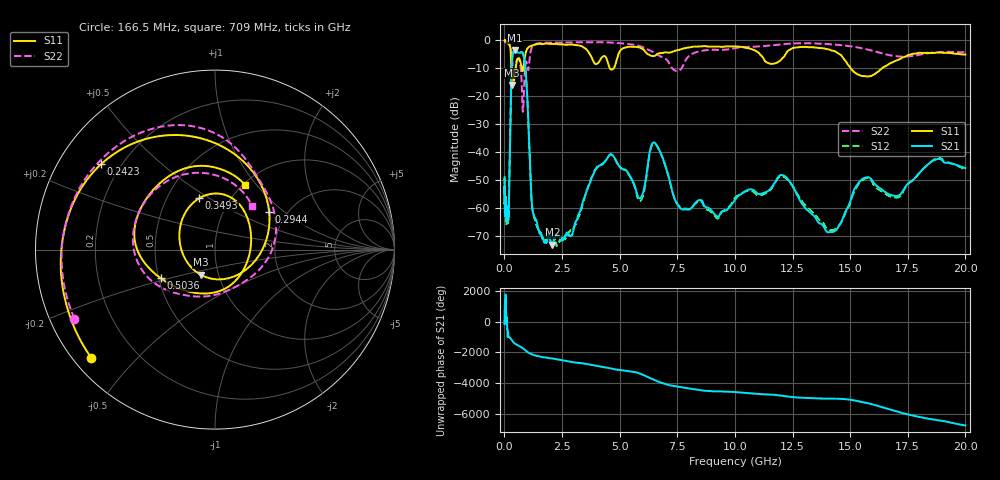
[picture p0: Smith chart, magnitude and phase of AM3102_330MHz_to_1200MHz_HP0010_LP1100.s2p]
! Date/Time: Tue, Sep 11, 2018 5:11 PM
! Network Analyzer: Agilent Technologies E8362B Rev: A.07.50.63
! Sweep from 0.010 to 20.000 GHz, 1601 Points, Sweep Type: LOG
! Power Supply: 4.949 V, 0.001 A
# Hz S DB R 50
!freq MagS11 AngS11 MagS21 AngS21 MagS12 AngS12 MagS22 AngS22
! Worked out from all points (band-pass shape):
!   1601 points, 10 MHz to 20 GHz, reference 50 ohm
!   highest |S21| = -3.37 dB at 458 MHz (marker M1); lowest = -73.0 dB at 2.084 GHz (marker M2)
!   |S21| within 3 dB of the highest: 338.8 MHz to 858 MHz (519.2 MHz wide, 86.8 % of centre)
!   lowest |S11| = -15.8 dB at 319.2 MHz (marker M3), VSWR 1.38, Z = 41.1 - j11.9 ohm
!   |S11| at or under -10 dB: 298 MHz to 495.4 MHz (197.4 MHz wide, 49.7 % of centre); 4.58 GHz to 4.735 GHz (154.1 MHz wide, 3.31 % of centre); 15.03 GHz to 16.37 GHz (1.347 GHz wide, 8.58 % of centre)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
!   |S22| runs from -25.5 to -0.3 dB; largest |S21 - S12| = 0.012
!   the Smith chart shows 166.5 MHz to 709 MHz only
!   S11 on the Smith chart (normalised r, x): 166.5 MHz: 0.05, -0.38; 242.3 MHz: 0.13, +0.33; 294.4 MHz: 1.63, +0.79; 349.3 MHz: 0.72, +0.45; 503.6 MHz: 0.51, -0.19; 709 MHz: 1.02, +0.87
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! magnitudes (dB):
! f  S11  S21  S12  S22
! 10 MHz  0.0  -49.3  -48.8  -0.3
! 35.55 MHz  0.0  -59.1  -60.4  -0.5
! 126.4 MHz  -0.4  -63.6  -60.6  -1.0
! 166.5 MHz  -0.8  -63.6  -63.2  -1.2
! 242.3 MHz  -2.0  -36.6  -36.6  -1.8
! 294.4 MHz  -8.7  -14.5  -14.6  -3.5
! 319.2 MHz  -15.8  -8.4  -8.4  -5.8
! 349.3 MHz  -10.5  -5.7  -5.8  -7.9
! 447.2 MHz  -13.0  -3.4  -3.4  -11.7
! 458 MHz  -12.5  -3.4  -3.4  -11.3
! 503.6 MHz  -9.3  -3.5  -3.7  -8.9
! 709 MHz  -8.0  -4.2  -4.3  -9.9
! 806 MHz  -10.7  -4.6  -4.7  -25.4
! 1.207 GHz  -1.8  -59.7  -59.7  -2.3
! 1.59 GHz  -1.3  -69.0  -69.0  -0.9
! 2.084 GHz  -1.2  -73.0  -70.2  -0.7
! 5.652 GHz  -2.3  -52.0  -52.3  -1.6
! 6.549 GHz  -5.4  -36.7  -36.9  -4.6
! 7.734 GHz  -2.9  -60.3  -60.0  -9.3
! 12.09 GHz  -6.1  -48.2  -48.6  -1.3
! 14.07 GHz  -3.2  -68.5  -67.5  -1.3
! 20 GHz  -5.0  -45.6  -46.2  -4.2
